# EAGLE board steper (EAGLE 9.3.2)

No outline drawn. Coordinates in mm, seen from the top.
Copper layers (1*16): Top 0.035mm / dielectric 1.5mm / Bottom 0.035mm
Design rules "default": minimum track width 6mil, minimum drill 0.35mm, track to track 6mil, track to pad 6mil, pad to pad 6mil, via to via 6mil, smd to smd 6mil, copper to edge 40mil, drill to drill 6mil, minimum pad ring 10mil, minimum via ring 8mil, stop-mask expansion 4mil, vias tented up to drill 0mil, thermal gap 10mil

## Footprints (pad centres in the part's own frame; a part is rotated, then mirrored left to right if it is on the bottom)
C2.5-2 = drill 0.813 pad 1.6 octagon: 1 -1.27,0; 2 1.27,0
CAPC3216X178N = smd 1.118 x 1.803: 1 -1.499,0; 2 1.499,0
1206 = smd 1.6 x 1.8: 1 -1.4,0; 2 1.4,0
1X4-SMT = smd 1.27 x 2.54: 1 -3.81,0; 2 -1.27,0; 3 1.27,0; 4 3.81,0
CSM-7X-DU = smd 5.5 x 2: 1 -4.75,0; 2 4.75,0
TQFP32-08THIN = smd 1.118 x 0.356: 1 -4.369,2.8; 8 -4.369,-2.8; 17 4.369,-2.8; 24 4.369,2.8 | smd 1.27 x 0.356: 2 -4.293,2; 3 -4.293,1.2; 4 -4.293,0.4; 5 -4.293,-0.4; 6 -4.293,-1.2; 7 -4.293,-2; 18 4.293,-2; 19 4.293,-1.2; 20 4.293,-0.4; 21 4.293,0.4; 22 4.293,1.2; 23 4.293,2 | smd 0.356 x 1.118: 9 -2.8,-4.369; 16 2.8,-4.369; 25 2.8,4.369; 32 -2.8,4.369 | smd 0.356 x 1.27: 10 -2,-4.293; 14 1.2,-4.293; 15 2,-4.293; 26 2,4.293; 27 1.2,4.293; 31 -2,4.293 | smd 0.35 x 1.27: 11 -1.2,-4.293; 12 -0.4,-4.293; 13 0.4,-4.293; 28 0.4,4.293; 29 -0.4,4.293; 30 -1.2,4.293
SOT223 = smd 1.499 x 2.007: 1 -2.261,-3.15; 2 0.025,-3.15; 3 2.311,-3.15 | smd 3.81 x 2.007: 4 0,3.15
SPC4078 = drill 0.8 pad 2.184 long: 1 -3,0; 2 0,-4.8 | drill 1 pad 2.184 long: 3 3,0
1X06_SMT = smd 1 x 2.5: 1 -6.35,1.52; 2 -3.81,-1.52; 3 -1.27,1.52; 4 1.27,-1.52; 5 3.81,1.52; 6 6.35,-1.52
1X13_SMT = smd 1 x 2.5: 1 -15.24,1.52; 2 -12.7,-1.52; 3 -10.16,1.52; 4 -7.62,-1.52; 5 -5.08,1.52; 6 -2.54,-1.52; 7 0,1.52; 8 2.54,-1.52; 9 5.08,1.52; 10 7.62,-1.52; 11 10.16,1.52; 12 12.7,-1.52; 13 15.24,1.52
P-LCC-4-3 = smd 1.1 x 1.5: A -0.8,1.5; B 0.8,1.5; G 0.8,-1.5; R -0.8,-1.5
0603 = smd 1.1 x 1: 1 -0.85,0; 2 0.85,0
TACTILE_SWITCH_SMD_4.6X2.8MM = smd 0.9 x 1: 1 -2.05,-0.8; 2 2.05,-0.8; 3 2.05,0.8; 4 -2.05,0.8
2X03SMD = smd 2.54 x 1.27: 1 -2.54,2.54; 2 2.92,2.54; 3 -2.54,0; 4 2.92,0; 5 -2.54,-2.54; 6 2.92,-2.54
1X06SMD = smd 2.54 x 1.27: 1 0,6.35; 2 0,3.81; 3 0,1.27; 4 0,-1.27; 5 0,-3.81; 6 0,-6.35
A4988BREAKOUT = drill 0.9: 1A 8.89,1.27; 1B 11.43,1.27; 2A 6.35,1.27; 2B 3.81,1.27; DIR 16.51,-11.43; EN -1.27,-11.43; GND 16.51,1.27; GND@0 1.27,1.27; MS1 1.27,-11.43; MS2 3.81,-11.43; MS3 6.35,-11.43; RST 8.89,-11.43; SLP 11.43,-11.43; STEP 13.97,-11.43; VDD 13.97,1.27; VMOT -1.27,1.27

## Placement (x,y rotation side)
C1  [C2.5-2]  -33.02,46.99 0 top
C2  22pF  [CAPC3216X178N]  -31.75,2.54 0 top
C3  22pF  [CAPC3216X178N]  -15.24,33.02 0 top
C6  10uF  [1206]  -45.72,48.26 0 top
C7  1uF  [1206]  -50.8,48.26 0 top
C8  100nF  [1206]  -15.24,55.88 0 top
CN1  1X4SMT  [1X4-SMT]  -30.48,54.61 0 top
CRYSTAL  16Mhz  [CSM-7X-DU]  -30.48,33.02 0 top
IC1  ATMEGA88-THIN  [TQFP32-08THIN]  -29.21,19.05 0 top
IC2  REG1117  [SOT223]  -49.53,3.81 0 top
J1  [SPC4078]  -62.23,3.81 0 top
JP1  [1X06_SMT]  -21.59,48.26 0 top
JP2  [1X13_SMT]  -30.48,40.64 0 top
LED1  [P-LCC-4-3]  -41.91,33.02 0 top
R1  10k  [0603]  -20.32,54.61 0 top
R2  10K  [0603]  -24.13,54.61 0 top
S1  [TACTILE_SWITCH_SMD_4.6X2.8MM]  -39.37,46.99 0 top
U$1  AVRISPSMD  [2X03SMD]  -39.37,5.08 0 top
U$2  FTDI-SMD-HEADER  [1X06SMD]  -30.48,-2.54 90 top
U$4  A4988BREAKOUT  [A4988BREAKOUT]  -15.24,8.89 0 top

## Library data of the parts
C1 = capacitor-wima
C2 C3 = AVX_By_element14_Batch_1; MPN: 0612ZC225MAT2A; OC_FARNELL: -; OC_NEWARK: 12N3209; SUPPLIER: AVX; TOLERANCE: ±20%; VOLTAGERATING: 10V
C6-C8 = 01_SparkFun
CN1 = adafruit
CRYSTAL = 01_FAB_Hello; OC_FARNELL: unknown; OC_NEWARK: unknown
IC1 LED1 U$1 U$2 = fab
IC2 = burr-brown; MPN: REG1117; OC_FARNELL: 1097566; OC_NEWARK: 14P6981
J1 = con-jack; OC_FARNELL: unknown; OC_NEWARK: unknown
JP1 JP2 = smd_con
R1 = SparkFun-Resistors; PROD_ID: RES-00824
R2 = SparkFun-Resistors; PROD_ID: RES-08269
S1 = SparkFun-Switches; PROD_ID: SWCH-13065
U$4 = RepRapjr

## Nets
12V: C1.1 IC2.3 J1.3 U$4.VMOT
CTS: IC1.19 U$2.2
GND: C1.2 C2.1 C3.1 C6.2 C7.2 C8.2 IC1.3 IC1.5 IC1.21 IC2.1 J1.1 J1.2 JP1.1 JP1.3 JP1.5 R1.1 S1.3 S1.4 U$1.6 U$2.1 U$4.GND U$4.GND@0
IN1: IC1.24 JP2.1
IN2: IC1.25 JP2.2
IN3: IC1.26 JP2.3
IN4: IC1.27 JP2.4
IN5: IC1.32 JP2.5
IN6: IC1.1 JP2.6
LED: IC1.23 LED1.A
MISO: IC1.16 U$1.1
MOSI: IC1.15 U$1.4
N$1: U$4.STEP
N$2: U$4.DIR
N$3: CN1.1 U$4.2B
N$4: CN1.2 U$4.2A
N$5: CN1.3 U$4.1A
N$6: CN1.4 U$4.1B
N$18: LED1.G R1.2
ON1: IC1.2 JP2.13
ON2: IC1.9 JP2.12
ON3: IC1.10 JP2.11
ON4: IC1.11 JP2.10
ON5: IC1.12 JP2.9
ON6: IC1.13 JP2.8
RESET: IC1.29 R2.1 S1.1 S1.2
RST: U$1.5
RTS: IC1.22 U$2.6
RX: IC1.30 U$2.5
SCK: IC1.17
SCL: IC1.28 U$1.3
SS: IC1.14 JP2.7
TX: IC1.31 U$2.4
VCC: C6.1 C7.1 C8.1 IC1.4 IC1.6 IC1.18 IC2.2 JP1.2 JP1.4 JP1.6 R2.2 U$1.2 U$2.3 U$4.VDD
XTAL1: C2.2 CRYSTAL.2 IC1.7
XTAL2: C3.2 CRYSTAL.1 IC1.8

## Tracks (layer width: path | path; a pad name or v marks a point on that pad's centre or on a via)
12V  (3 unrouted)
CTS  (1 unrouted)
GND  (21 unrouted)
IN1  (1 unrouted)
IN2  (1 unrouted)
IN3  (1 unrouted)
IN4  (1 unrouted)
IN5  (1 unrouted)
IN6  (1 unrouted)
LED  (1 unrouted)
MISO  (1 unrouted)
MOSI  (1 unrouted)
N$3  (1 unrouted)
N$4  (1 unrouted)
N$5  (1 unrouted)
N$6  (1 unrouted)
N$18  (1 unrouted)
ON1  (1 unrouted)
ON2  (1 unrouted)
ON3  (1 unrouted)
ON4  (1 unrouted)
ON5  (1 unrouted)
ON6  (1 unrouted)
RESET  (3 unrouted)
RTS  (1 unrouted)
RX  (1 unrouted)
SCL  (1 unrouted)
SS  (1 unrouted)
TX  (1 unrouted)
VCC  (13 unrouted)
XTAL1  (2 unrouted)
XTAL2  (2 unrouted)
